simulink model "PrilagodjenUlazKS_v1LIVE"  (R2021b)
settings: Solver=VariableStepAuto  StartTime=0.0  StopTime=200e-09  MaxStep=0.05e-09  RelTol=1e-3
libraries: fl_lib x10, nesl_utility x5, simulink x1, ee_lib x1

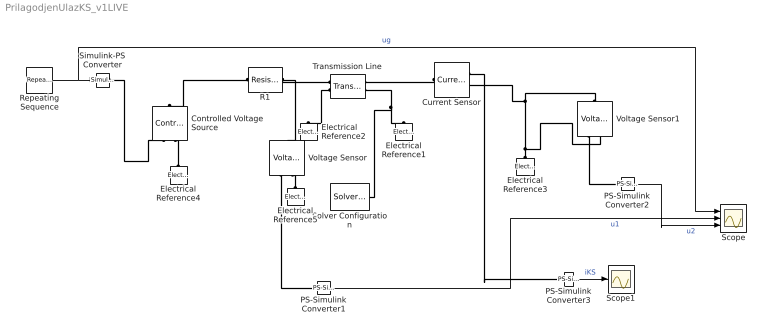
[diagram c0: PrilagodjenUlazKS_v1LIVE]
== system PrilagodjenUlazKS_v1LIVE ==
  Controlled Voltage Source : fl_lib/Electrical/Electrical Sources/Controlled Voltage Source
  Current Sensor : fl_lib/Electrical/Electrical Sensors/Current Sensor
  Electrical Reference{1..5} (5 alike) : fl_lib/Electrical/Electrical Elements/Electrical Reference
  PS-Simulink Converter1 : nesl_utility/PS-Simulink Converter  PhysicalDomain=network_engine_domain  SubClassName=ps_output  LeftPortType=input  RightPortType=output  PseudoPeriodic=off  Frequencies=[]  Unit=inherit  AffineConversion=off
  PS-Simulink Converter2 : nesl_utility/PS-Simulink Converter  PhysicalDomain=network_engine_domain  SubClassName=ps_output  LeftPortType=input  RightPortType=output  PseudoPeriodic=off  Frequencies=[]  Unit=inherit  AffineConversion=off
  PS-Simulink Converter3 : nesl_utility/PS-Simulink Converter  PhysicalDomain=network_engine_domain  SubClassName=ps_output  LeftPortType=input  RightPortType=output  PseudoPeriodic=off  Frequencies=[]  Unit=inherit  AffineConversion=off
  R1 : fl_lib/Electrical/Electrical Elements/Resistor  R=50 Ohm  i_specify=off  i_priority=None  i=0 A  i_nominal_specify=off  i_nominal_unit=A  i_nominal_value=1  v_specify=off  v_priority=None  v=0 V  v_nominal_specify=off  v_nominal_unit=V  v_nominal_value=1
  Repeating Sequence : simulink/Sources/Repeating Sequence  rep_seq_t=[0 1 20 21 300]*1e-9  rep_seq_y=[0 1 1 0 0]
  Scope : Scope  NumInputPorts=3
  Scope1 : Scope
  Simulink-PS Converter : nesl_utility/Simulink-PS Converter  PhysicalDomain=network_engine_domain  SubClassName=ps_input  LeftPortType=input  RightPortType=output  PseudoPeriodic=off  Frequencies=[]  NoiseDistribution=none  NoiseParameters=[]  Unit=1  AffineConversion=off  FilteringAndDerivatives=provide  SimscapeFilterOrder=1  InputFilterTimeConstant=0.001  UdotUserProvided=0
  Solver Configuration : nesl_utility/Solver Configuration  PhysicalDomain=network_engine_domain  SubClassName=solver  LeftPortType=input  RightPortType=generic  Tones=[]  Harmonics=[]  SimulateNoise=off  Profile=off  UseLocalSampling=off  EnableSwitchedLinearOptims=on  FrequencyDomain=off  UseCCode=off  RelTol=0.001  AbsTol=1e-06  MinStep=1e-09  ToWorkspace=off  RevertToSquareIcSolve=off  NumHomotopyIterations=100  PhasorMode=off  PhasorModeNumHarmonics=1  DoDC=off  ResidualTolerance=1e-09  UseLocalSolver=off  LocalSolverChoice=NE_BACKWARD_EULER_ADVANCER  LocalSolverSampleTime=0.001  DoFixedCost=off  MaxNonlinIter=3  MaxModeIter=2  ComputeImpulses=off  ImpulseIterations=2  LinearAlgebra=auto  EquationFormulation=NE_TIME_EF  DelaysMemoryBudget=1024  AutomaticFiltering=on  FilteringTimeConstant=0.001  PartitionStorageMethod=AS_NEEDED  PartitionMemoryBudget=1024  PartitionMethod=ROBUST
  Transmission Line : ee_lib/Passive/Lines/Transmission Line  model_type=1  TD=60 ns  LC_param=1  Z0_delay_based=50 Ohm  Z0=50 Ohm  freq=60 Hz  Ll=220 uH/m  L=220 uH/m  C=90 pF/m  R=0.3 Ohm/m  G=5e-6 S/m  LEN=1 m  N=1
  Voltage Sensor : fl_lib/Electrical/Electrical Sensors/Voltage Sensor
  Voltage Sensor1 : fl_lib/Electrical/Electrical Sensors/Voltage Sensor
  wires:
  Repeating Sequence/1 -> Scope/1, Simulink-PS Converter/1  "ug"
  PS-Simulink Converter1/1 -> Scope/2  "u1"
  PS-Simulink Converter2/1 -> Scope/3  "u2"
  PS-Simulink Converter3/1 -> Scope1/1  "iKS"
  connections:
  R1/RConn1 -- Transmission Line/LConn1 -- Voltage Sensor/LConn1
  Voltage Sensor1/LConn1 -- Current Sensor/RConn2 -- Voltage Sensor1/RConn2 -- Electrical Reference3/LConn1
  Transmission Line/LConn2 -- Electrical Reference2/LConn1
  Transmission Line/RConn2 -- Solver Configuration/RConn1 -- Electrical Reference1/LConn1
  R1/LConn1 -- Controlled Voltage Source/LConn1
  Electrical Reference4/LConn1 -- Controlled Voltage Source/RConn2
  Simulink-PS Converter/RConn1 -- Controlled Voltage Source/RConn1
  Electrical Reference5/LConn1 -- Voltage Sensor/RConn2
  Voltage Sensor/RConn1 -- PS-Simulink Converter1/LConn1
  Voltage Sensor1/RConn1 -- PS-Simulink Converter2/LConn1
  Current Sensor/LConn1 -- Transmission Line/RConn1
  Current Sensor/RConn1 -- PS-Simulink Converter3/LConn1
